FUNCTION_BLOCK FB104
TITLE =Set Object
//********************************************************************************
//* maxon motor ag
//* R&D
//* all rights reserved
//********************************************************************************
//* Summary:  Writes one object from object dictionary
//*
//* Remarks:
//*
//* Created under: STEP7 REV5.2+SP1
//********************************************************************************
//* History:
//* 25.05.2004 | ina   first release
//*
//*
//********************************************************************************
//

AUTHOR:INA
FAMILY:Utilitie
NAME:SObject
VERSION:00.01


VAR_INPUT

Write : BOOL //A rising edge start the command

  NodeID : BYTE //Adress of the maxon device

  ObjectIndex : WORD //Index

  ObjectSubIndex : BYTE //Subindex

  Length : BYTE //Length in bytes

  Data : DINT //Data

END_VAR
VAR_OUTPUT
  Done : BOOL //Data valid flag is TRUE if data were available

  Err : BOOL //Error flag is TRUE if an

  ErrNo : DINT //Contains detailed error information

END_VAR
VAR
  xEdgeMerker : BOOL //Edge Merker

  xEdgeFlag : BOOL //Edge Flag

  xStep : INT //State variable

  xObjectIndex : DWORD
  xObjectSubIndex : DWORD
  xDataByte : BYTE
  xDataWord : WORD
  xDataDWord : DWORD
  xDataChar : CHAR
END_VAR

BEGIN

NETWORK
TITLE = Activat the service function
//

// SDO Write "Set Object"

       U    #Write
       FP   #xEdgeFlag                   // recognize a positiv edge of the Read signal
       =    #xEdgeMerker                 // and set the xEdgeMerker for one cycle to true

       L    #xStep
       L    0
       ==I
       U    #xEdgeMerker
       SPB  nstp                         // iStep = 1 -> fnc1

       L    #xStep                       // jump list
       SPL  List
       SPA  rdef
       SPA  fnc1
       SPA  fncE
List  :SPA  rdef

rdef  :NOP  0                            // redefine the done signal
       R    #Done                        // reset Done
       L    0
       T    #xStep                       // iStep = 0
       SPA  end

fnc1  :NOP  0
       L    #ObjectIndex
       T    #xObjectIndex

       L    #ObjectSubIndex
       T    #xObjectSubIndex

       L    #Length
       L    1
       ==I
       SPB  one

       L    #Length
       L    2
       ==I
       SPB  two
       SPA  four

one   :NOP  0
       L    #Data
       T    #xDataByte
       T    #xDataChar

       CALL FC14
         NodeID:=#NodeID
         Index:=#xObjectIndex
         SubIndex:=#xObjectSubIndex
         ValueIn:=#xDataByte
         RET_VAL:=#Done
         Err:=#Err
         ErrNo:=#ErrNo

       SPA  fncE                         // iStep = 2 -> fncE

two   :NOP  0
       L    #Data
       T    #xDataWord

       CALL FC15
         NodeID:=#NodeID
         Index:=#xObjectIndex
         SubIndex:=#xObjectSubIndex
         ValueIn:=#xDataWord
         RET_VAL:=#Done
         Err:=#Err
         ErrNo:=#ErrNo

       SPA  fncE                         // iStep = 2 -> fncE

four  :NOP  0
       L    #Data
       T    #xDataDWord

       CALL FC16
         NodeID:=#NodeID
         Index:=#xObjectIndex
         SubIndex:=#xObjectSubIndex
         ValueIn:=#xDataDWord
         RET_VAL:=#Done
         Err:=#Err
         ErrNo:=#ErrNo

       SPA  fncE                         // iStep = 2 -> fncE

fncE  :NOP  0
       L    0
       T    #xStep
       SPA  end

nstp  :NOP  0
       L    #xStep
       INC            1
       T    #xStep

end   :NOP  0
END_FUNCTION_BLOCK
